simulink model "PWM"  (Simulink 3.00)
settings: Solver=ode45  StartTime=0.0  StopTime=100.0  RelTol=1e-3

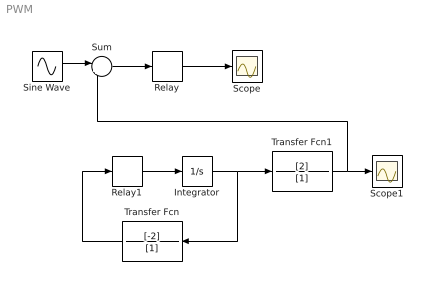
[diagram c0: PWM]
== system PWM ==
  Integrator : Integrator  ExternalReset=none  InitialConditionSource=internal  InitialCondition=0.05  LimitOutput=off  UpperSaturationLimit=inf  LowerSaturationLimit=-inf  ShowSaturationPort=off  ShowStatePort=off  AbsoluteTolerance=auto
  Relay : Relay  OnSwitchValue=0.1  OffSwitchValue=-0.1  OnOutputValue=1  OffOutputValue=-1
  Relay1 : Relay  OnSwitchValue=1  OffSwitchValue=-1  OnOutputValue=1  OffOutputValue=-1
  Scope : Scope
  Scope1 : Scope
  Sine Wave : Sin  Amplitude=1  Frequency=.2  Phase=0  SampleTime=0
  Sum : Sum  Inputs=|+-  SaturateOnIntegerOverflow=on
  Transfer Fcn : TransferFcn  Orientation=left  Numerator=[-2]  Denominator=[1]
  Transfer Fcn1 : TransferFcn  Numerator=[2]  Denominator=[1]
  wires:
  Sum/1 -> Relay/1
  Relay/1 -> Scope/1
  Sine Wave/1 -> Sum/1
  Relay1/1 -> Integrator/1
  Integrator/1 -> Transfer Fcn/1, Transfer Fcn1/1
  Transfer Fcn/1 -> Relay1/1
  Transfer Fcn1/1 -> Scope1/1, Sum/2
